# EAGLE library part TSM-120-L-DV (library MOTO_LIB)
.100" (2.54mm) Surface Mount, 2x20 Double Row, Vertical Mount, Male
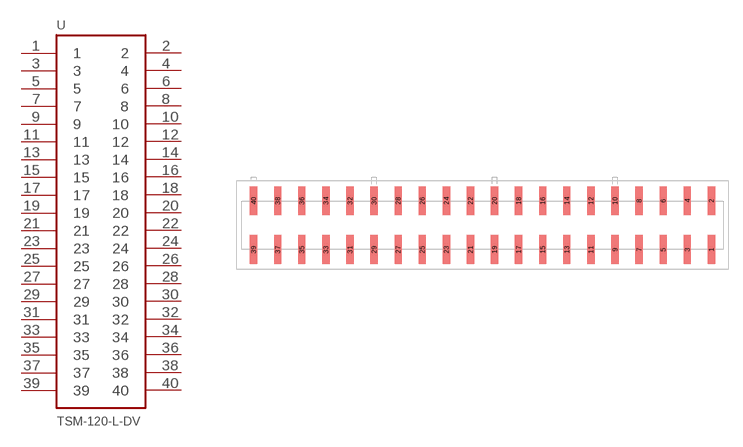
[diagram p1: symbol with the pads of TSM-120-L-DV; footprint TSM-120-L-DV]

Designator prefix -

## TSM-120-L-DV (MPN: ASP-193073-01; SUPPLIER: SAMTEC)  [TSM-120-L-DV]
1  1
2  2
3  3
4  4
5  5
6  6
7  7
8  8
9  9
10  10
11  11
12  12
13  13
14  14
15  15
16  16
17  17
18  18
19  19
20  20
21  21
22  22
23  23
24  24
25  25
26  26
27  27
28  28
29  29
30  30
31  31
32  32
33  33
34  34
35  35
36  36
37  37
38  38
39  39
40  40

## Footprint TSM-120-L-DV (pad centres in mm)
.100" (2,54mm) Surface Mount, Double Row, Vertical Mount. manufacturer:SAMTEC
smd 0.77 x 3.041: 1 24.13,-2.577; 2 24.13,2.577; 3 21.59,-2.577; 4 21.59,2.577; 5 19.05,-2.577; 6 19.05,2.577; 7 16.51,-2.577; 8 16.51,2.577; 9 13.97,-2.577; 10 13.97,2.577; 11 11.43,-2.577; 12 11.43,2.577; 13 8.89,-2.577; 14 8.89,2.577; 15 6.35,-2.577; 16 6.35,2.577; 17 3.81,-2.577; 18 3.81,2.577; 19 1.27,-2.577; 20 1.27,2.577; 21 -1.27,-2.577; 22 -1.27,2.577; 23 -3.81,-2.577; 24 -3.81,2.577; 25 -6.35,-2.577; 26 -6.35,2.577; 27 -8.89,-2.577; 28 -8.89,2.577; 29 -11.43,-2.577; 30 -11.43,2.577; 31 -13.97,-2.577; 32 -13.97,2.577; 33 -16.51,-2.577; 34 -16.51,2.577; 35 -19.05,-2.577; 36 -19.05,2.577; 37 -21.59,-2.577; 38 -21.59,2.577; 39 -24.13,-2.577; 40 -24.13,2.577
